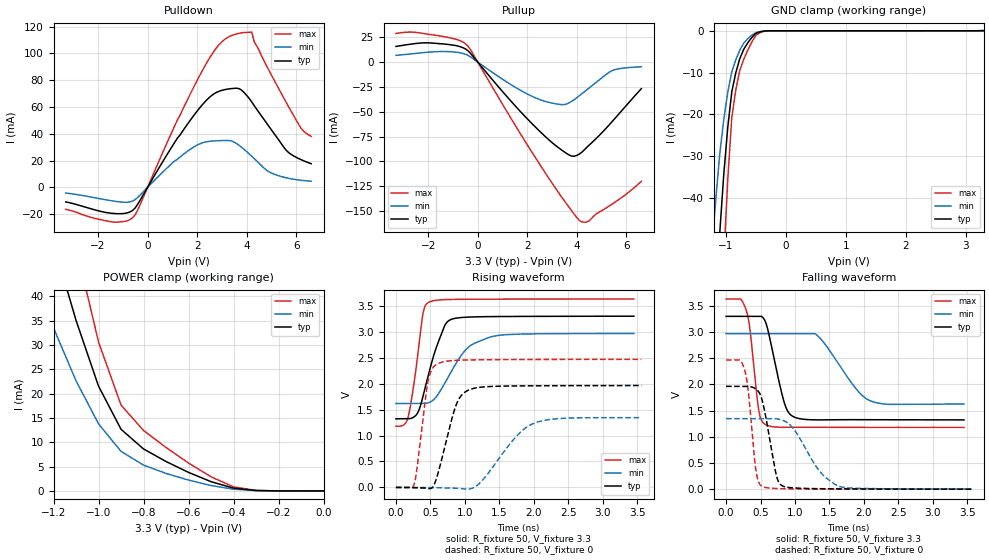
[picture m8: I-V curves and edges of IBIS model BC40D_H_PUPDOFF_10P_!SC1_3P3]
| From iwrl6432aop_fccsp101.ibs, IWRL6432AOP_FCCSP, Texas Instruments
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|   Model Cell BC40D_H_PUPDOFF_10P_!SC1_3P3
|BC40D_H_PUPDOFF_10P_!SC1_3P3
[Model]   BC40D_H_PUPDOFF_10P_!SC1_3P3
Model_type   I/O
Polarity   Non-Inverting
Enable   Active-Low
Vinl =  0.8V
Vinh =  2V
Cref =  15pF
Rref =  100.0000M
Vref =  0V
Vmeas =  1.65
C_comp   2.157014p   1.997104p   2.250886p
|[Input load] weak_pupdoff
|[Output drive] fast
|[supplytol] 10
|[temp] ind
[Model Spec]
Vinl   0.8V   0.8V   0.8V
Vinh   2V   2V   2V
[Temperature Range]   25   125   -40
[Voltage Range]   3.3   2.97   3.63
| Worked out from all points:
|   slope of the pulldown table from 0 to 0.495 V, typ, clamps not added: 31.8 ohm
|   slope of the pullup table from 0 to 0.495 V, typ, clamps not added: 33.3 ohm
|   GND clamp passes 1 mA (typ) near -0.53 V on its own axis
|   POWER clamp passes 1 mA (typ) near -0.43 V on its own axis
|   rising waveform, R_fixture 50, V_fixture 3.3: 20-80 % time 258ps typ, 390ps min, 146ps max; typ from 1.32 V to 3.3 V
|   rising waveform, R_fixture 50, V_fixture 0: 20-80 % time 233ps typ, 479ps min, 138ps max; typ from 0 V to 1.96 V
|   falling waveform, R_fixture 50, V_fixture 3.3: 20-80 % time 199ps typ, 427ps min, 119ps max; typ from 3.3 V to 1.32 V
|   falling waveform, R_fixture 50, V_fixture 0: 20-80 % time 162ps typ, 386ps min, 107ps max; typ from 1.96 V to 0 V
| Nom Voltages:
|   VDD=1.1001, VDDS=3.3, VDDS18=1.8, ESD_BIASFET=0, VSS=0, VSSS=0
| Min Voltages:
|   VDD=0.99, VDDS=2.97, VDDS18=1.62, ESD_BIASFET=0, VSS=0, VSSS=0
| Max Voltages:
|   VDD=1.21, VDDS=3.63, VDDS18=1.98, ESD_BIASFET=0, VSS=0, VSSS=0
[POWER_clamp]
|   voltage   I(typ)   I(min)   I(max)
-3.3V     446.9mA    419.5mA    603.9mA
-1.267V   62.17mA    41.5mA     88.03mA
-1.233V   56.52mA    37.5mA     80.22mA
-1.133V   40.34mA    26.27mA    57.61mA
-1.067V   30.56mA    19.7mA     43.68mA
-1.033V   26.05mA    16.75mA    37.15mA
-1V       21.55mA    13.8mA     30.62mA
-900mV    12.68mA    8.135mA    17.65mA
-800mV    8.63mA     5.309mA    12.43mA
-600mV    3.813mA    2.231mA    5.733mA
-400mV    580.7uA    357.1uA    842.6uA
0V        4.589uA    2.01uA     9.301uA
[Pulldown]
|   voltage   I(typ)   I(min)   I(max)
-3.3V     -10.92mA   -4.307mA   -16.45mA
-1.4V     -19.52mA   -10.22mA   -25.94mA
-600mV    -17.22mA   -10.25mA   -22.66mA
1.1V      33.8mA     19.88mA    46.22mA
2.1V      59.3mA     32.44mA    83.48mA
2.9V      71.86mA    34.84mA    107mA
3.5V      73.95mA    33.66mA    114.2mA
4.2V      63.8mA     23.19mA    116mA
4.9V      45.33mA    11.53mA    87.2mA
5.6V      27.47mA    7.046mA    63.1mA
6.2V      20.56mA    5.221mA    43.87mA
6.6V      17.6mA     4.555mA    38.05mA
[Pullup]
|   voltage   I(typ)   I(min)   I(max)
-3.3V     15.77mA    6.741mA    28.8mA
-1.9V     19.23mA    10.15mA    27.67mA
-900mV    16.69mA    10.02mA    23.17mA
-400mV    11.53mA    6.853mA    16.25mA
1.3V      -38.16mA   -22.04mA   -54.89mA
2.3V      -64.7mA    -35.66mA   -95.04mA
3.4V      -88.76mA   -42.82mA   -136.4mA
3.8V      -94.64mA   -39.36mA   -150mA
4.1V      -92.52mA   -33.79mA   -159.3mA
4.4V      -85.77mA   -27.94mA   -161mA
5.4V      -60.46mA   -8.849mA   -143.2mA
6.6V      -26.71mA   -4.741mA   -120mA
[GND_clamp]
|   voltage   I(typ)   I(min)   I(max)
-3.3V     -787.2mA   -607.8mA   -1.235A
-1.233V   -85.66mA   -52.14mA   -138.8mA
-1.167V   -66.47mA   -40.37mA   -107.7mA
-1.1V     -48.25mA   -29.37mA   -77.98mA
-1.033V   -34.27mA   -21.19mA   -54.56mA
-966.7mV  -23.06mA   -14.66mA   -35.51mA
-900mV    -14.61mA   -9.789mA   -20.83mA
-833.3mV  -10.05mA   -6.934mA   -14.15mA
-700mV    -4.416mA   -2.931mA   -6.81mA
-500mV    -621.6uA   -443.4uA   -1.094mA
-300mV    -17.13uA   -24.29uA   -23.57uA
3.3V      4.589uA    110.6uA    5.608uA
[Ramp]
| variable   typ   min   max
dV/dt_f  1.1960336/0.20096935n 0.83589558/0.44374699n  1.4762162/0.11982334n
dV/dt_r  1.1926872/0.23597166n 0.82875311/0.49110066n  1.4908098/0.13892893n
R_load = 50
[Rising Waveform]
R_fixture = 50
V_fixture = 3.3
V_fixture_min = 2.97
V_fixture_max = 3.63
|   time   V(typ)   V(min)   V(max)
0s        1.323V     1.617V     1.18V
177.6ps   1.323V     1.617V     1.36V
304ps     1.412V     1.617V     2.412V
390.2ps   1.739V     1.617V     3.331V
475.7ps   2.192V     1.633V     3.568V
695ps     3.082V     1.975V     3.618V
826ps     3.249V     2.286V     3.623V
1.069ns   3.283V     2.721V     3.626V
1.437ns   3.293V     2.919V     3.628V
3.453ns   3.299V     2.966V     3.63V
[Rising Waveform]
R_fixture = 50
V_fixture = 0
V_fixture_min = 0
V_fixture_max = 0
|   time   V(typ)   V(min)   V(max)
0s        0V         0V         0V
263ps     -5.429mV   0V         55.93mV
302.5ps   -7.292mV   0V         330.3mV
465.3ps   -20.65mV   -2.402mV   2.039V
538ps     15.36mV    -3.759mV   2.309V
608ps     258.6mV    -5.575mV   2.384V
871.4ps   1.58V      -15.22mV   2.448V
1.058ns   1.877V     -31.71mV   2.456V
2.001ns   1.958V     1.235V     2.466V
3.562ns   1.963V     1.344V     2.468V
[Falling Waveform]
R_fixture = 50
V_fixture = 3.3
V_fixture_min = 2.97
V_fixture_max = 3.63
|   time   V(typ)   V(min)   V(max)
0s        3.299V     2.969V     3.629V
296.4ps   3.299V     2.969V     3.4V
344.8ps   3.299V     2.969V     3.075V
474.5ps   3.299V     2.969V     1.512V
574.9ps   3.184V     2.969V     1.231V
838.8ps   1.679V     2.969V     1.181V
978.7ps   1.383V     2.969V     1.181V
1.328ns   1.322V     2.931V     1.181V
2.098ns   1.325V     1.685V     1.179V
3.453ns   1.322V     1.625V     1.179V
[Falling Waveform]
R_fixture = 50
V_fixture = 0
V_fixture_min = 0
V_fixture_max = 0
|   time   V(typ)   V(min)   V(max)
0s        1.963V     1.347V     2.467V
272.9ps   1.963V     1.347V     2.261V
324.2ps   1.961V     1.347V     1.853V
432.9ps   1.912V     1.347V     366mV
521.1ps   1.711V     1.347V     54.35mV
729.9ps   264.7mV    1.344V     12.34mV
829.8ps   55.57mV    1.31V      7.312mV
1.374ns   7.945mV    315.5mV    0V
1.631ns   5.684mV    58.93mV    0V
3.562ns   0V         3.208mV    0V
